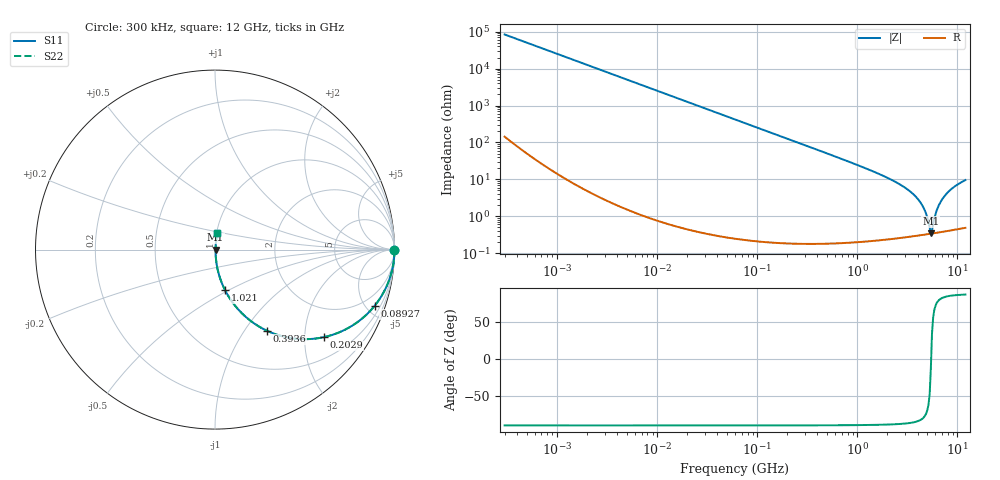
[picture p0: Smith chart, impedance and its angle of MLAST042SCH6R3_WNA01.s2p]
! MLAST042SCH6R3_WNA01  S-PARAMETER MODEL  ( General Type )
! Model Generated by TAIYO YUDEN Corporation (http://www.ty-top.com)
! Version 1.0
! TAIYO YUDEN Control No. 150820
! Copyright(c) 2015 TAIYO YUDEN CO.,LTD. All Rights Reserved.
! Product Description (link to TY-COMPAS)
! https://ds.yuden.co.jp/TYCOMPAS/or/detail?pn=MLAST042SCH6R3BWNA01&u=M
! Products Name : Multilayer Ceramic Capacitors
! Characteristics :
!  Capacitance : 6.3 pF , Rated Voltage : 25V , TCC : CH / C0H
!  Case Size : 0.4 x 0.2 / 0.016 x 0.008 [mm/inch] , Thickness : 0.2 / 0.008 [mm/inch]
!  (Conditions: Temperature = 25 degC , DC Bias Current/Voltage = 0A / 0V)
! External Node Assignments :
!  1  o---| |---o  2
! GND o---------o GND
! Frequency Range : 0.3MHz  -  12000MHz  [ 401 STEP ]
# MHz S RI R 50
! Freq[MHz].  S11 Real  S11 Imag  S21 Real  S21 Imag  S12 Real  S12 Imag  S22 Real  S22 Imag
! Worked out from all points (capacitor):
!   401 points, 300 kHz to 12 GHz, reference 50 ohm
!   read as one part in series: C = 6.28 pF near 316.3 kHz
!   lowest |Z| = 346 mohm at 5.42 GHz (marker M1)
!   series resonance near 5.458 GHz, so ESL is about 140 pH
!   S11 on the Smith chart (normalised r, x): 300 kHz: open; 89.27 MHz: 1.00, -5.67; 202.9 MHz: 1.00, -2.49; 393.6 MHz: 1.00, -1.28; 1.021 GHz: 1.00, -0.48; 12 GHz: 1.01, +0.19
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0.3  1 -0.00118  3.41e-06 0.00118  3.41e-06 0.00118  1 -0.00118
1.769972  0.9999 -0.00698  5.16e-05 0.00698  5.16e-05 0.00698  0.9999 -0.00698
10.44266  0.9983 -0.0411  0.00171 0.0411  0.00171 0.0411  0.9983 -0.0411
27.82928  0.988 -0.1085  0.012 0.1085  0.012 0.1085  0.988 -0.1085
60  0.9468 -0.2242  0.0532 0.2242  0.0532 0.2242  0.9468 -0.2242
89.27472  0.8893 -0.3133  0.1107 0.3133  0.1107 0.3133  0.8893 -0.3133
202.9496  0.6084 -0.4874  0.3916 0.4874  0.3916 0.4874  0.6084 -0.4874
353.9943  0.3373 -0.4715  0.6627 0.4715  0.6627 0.4715  0.3373 -0.4715
393.5654  0.2914 -0.453  0.7086 0.453  0.7086 0.453  0.2914 -0.453
617.4538  0.1421 -0.3469  0.8579 0.3469  0.8579 0.3469  0.1421 -0.3469
1021.415  0.0559 -0.2256  0.9441 0.2256  0.9441 0.2256  0.0559 -0.2256
2088.533  0.0129 -0.1022  0.9871 0.1022  0.9871 0.1022  0.0129 -0.1022
3026.31  0.00603 -0.0578  0.994 0.0578  0.994 0.0578  0.00603 -0.0578
3944.255  0.00391 -0.0309  0.9961 0.0309  0.9961 0.0309  0.00391 -0.0309
4623.766  0.00339 -0.0158  0.9966 0.0158  0.9966 0.0158  0.00339 -0.0158
5278.635  0.00333 -0.0036  0.9967 0.0036  0.9967 0.0036  0.00333 -0.0036
5420.343  0.00335 -0.00079  0.9966 0.00079  0.9966 0.00079  0.00335 -0.00079
5715.274  0.00345 0.00506  0.9965 -0.00506  0.9965 -0.00506  0.00345 0.00506
6354.153  0.00386 0.0164  0.9961 -0.0164  0.9961 -0.0164  0.00386 0.0164
7254.098  0.00482 0.0317  0.9952 -0.0317  0.9952 -0.0317  0.00482 0.0317
8966.534  0.00755 0.0577  0.9924 -0.0577  0.9924 -0.0577  0.00755 0.0577
12000  0.0138 0.0939  0.9862 -0.0939  0.9862 -0.0939  0.0138 0.0939
